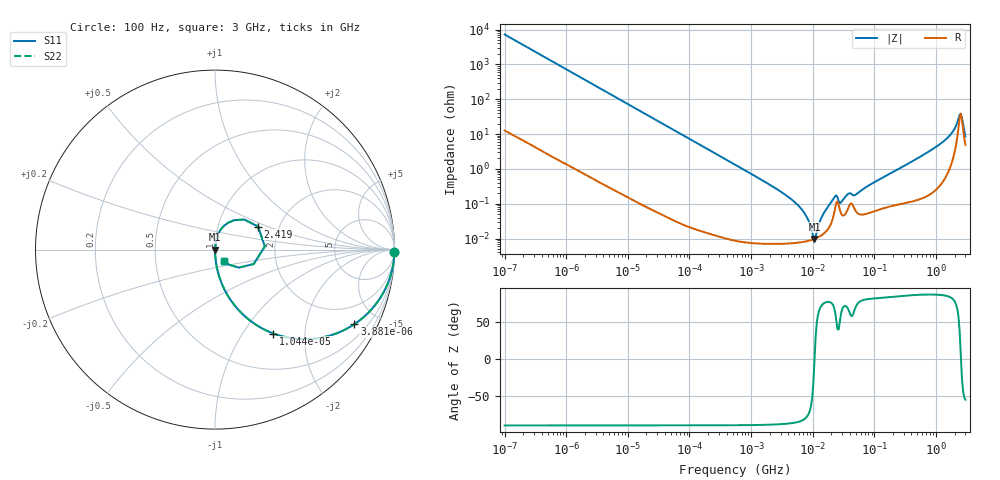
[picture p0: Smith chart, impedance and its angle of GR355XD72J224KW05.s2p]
!Murata Part Number: GR355XD72J224KW05
!These Parameters are Measured in Series Mode Connection
!Data Generated on Jan 08, 2026
!  o--ll--o
!Port1  Port2
!  o------o
!Operation Temp=25[degC], DC Bias Voltage=0[V]
!Freq. Start=100[Hz] Stop=3[GHz] 401[Steps]
# Hz S RI R 50
!Freq.(Hz) S11(Real) S11(Imag) S21(Real) S21(Imag) S12(Real) S12(Imag) S22(Real) S22(Imag)
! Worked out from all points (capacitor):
!   401 points, 100 Hz to 3 GHz, reference 50 ohm
!   read as one part in series: C = 221 nF near 109 Hz
!   lowest |Z| = 9.82 mohm at 10.67 MHz (marker M1)
!   series resonance near 10.69 MHz, so ESL is about 1 nH
!   S11 on the Smith chart (normalised r, x): 100 Hz: open; 3.881 kHz: 1.01, -3.73; 10.44 kHz: 1.00, -1.39; 2.419 GHz: 1.56, +0.43; 3 GHz: 1.10, -0.14
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100  0.9998 -0.0139  0.000217 0.0139  0.000217 0.0139  0.9998 -0.0139
536  0.9944 -0.0737  0.0056 0.0737  0.0056 0.0737  0.9944 -0.0737
1788  0.9421 -0.2327  0.0579 0.2327  0.0579 0.2327  0.9421 -0.2327
3881  0.7765 -0.4156  0.2235 0.4156  0.2235 0.4156  0.7765 -0.4156
10443  0.3257 -0.4676  0.6743 0.4676  0.6743 0.4676  0.3257 -0.4676
31977  0.0495 -0.2158  0.9505 0.2158  0.9505 0.2158  0.0495 -0.2158
547723  0.000263 -0.0133  0.9997 0.0133  0.9997 0.0133  0.000263 -0.0133
4919190  7.54e-05 -0.00118  0.9999 0.00118  0.9999 0.00118  7.54e-05 -0.00118
7565221  8.26e-05 -0.000488  0.9999 0.000488  0.9999 0.000488  8.26e-05 -0.000488
9794414  9.3e-05 -0.000122  0.9999 0.000122  0.9999 0.000122  9.3e-05 -0.000122
1.067491e7  9.82e-05 -1.9e-06  0.9999 1.9e-06  0.9999 1.9e-06  9.82e-05 -1.9e-06
1.506283e7  0.000139 0.000512  0.9999 -0.000512  0.9999 -0.000512  0.000139 0.000512
2.21892e7  0.000527 0.00139  0.9995 -0.00139  0.9995 -0.00139  0.000527 0.00139
2.872754e7  0.000531 0.000946  0.9995 -0.000946  0.9995 -0.000946  0.000531 0.000946
3.71925e7  0.000714 0.00175  0.9993 -0.00175  0.9993 -0.00175  0.000714 0.00175
5.026954e7  0.000608 0.00174  0.9994 -0.00174  0.9994 -0.00174  0.000608 0.00174
1.751444e8  0.000876 0.0071  0.9991 -0.0071  0.9991 -0.0071  0.000876 0.0071
1.214989e9  0.0066 0.0541  0.9934 -0.0541  0.9934 -0.0541  0.0066 0.0541
1.950712e9  0.0393 0.1208  0.9607 -0.1208  0.9607 -0.1208  0.0393 0.1208
2.419119e9  0.2399 0.1287  0.7601 -0.1287  0.7601 -0.1287  0.2399 0.1287
2.636591e9  0.2159 -0.0801  0.7841 0.0801  0.7841 0.0801  0.2159 -0.0801
3e9  0.051 -0.0636  0.949 0.0636  0.949 0.0636  0.051 -0.0636
